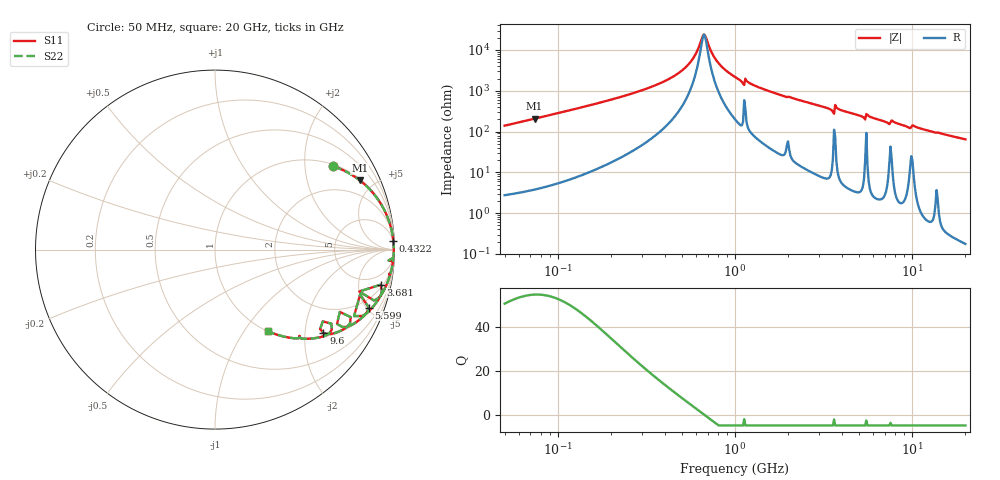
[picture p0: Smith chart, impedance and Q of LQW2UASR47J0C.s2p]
!Murata Part Number: LQW2UASR47J0C
!These Parameters are Measured in Series Mode Connection
!  o--[Z]--o
!Port1  Port2
!  o-------o
!Freq. Start=50[MHz] Stop=20[GHz], 401[Steps]
# Hz S RI R 50
!Freq.(Hz) S11(Real) S11(Imag) S21(Real) S21(Imag) S12(Real) S12(Imag) S22(Real) S22(Imag)
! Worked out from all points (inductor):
!   401 points, 50 MHz to 20 GHz, reference 50 ohm
!   read as one part in series: L = 442 nH near 51.52 MHz
!   highest Q = 54.7 at 73.81 MHz (marker M1), where L = 447 nH
!   self-resonance near 667.4 MHz
!   S11 on the Smith chart (normalised r, x): 50 MHz: 1.06, +2.79; 432.2 MHz: 5, +41; 3.681 GHz: 2.47, -8.87; 5.599 GHz: 1.30, -5.18; 9.6 GHz: 1.13, -2.49; 20 GHz: 1.00, -1.29
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5e7  0.6582 0.4646  0.3418 -0.4646  0.3418 -0.4646  0.6582 0.4646
7.380808e7  0.8069 0.3857  0.1931 -0.3857  0.1931 -0.3857  0.8069 0.3857
1.364002e8  0.9352 0.2357  0.0648 -0.2357  0.0648 -0.2357  0.9352 0.2357
3.721004e8  0.9913 0.0661  0.00867 -0.0661  0.00867 -0.0661  0.9913 0.0661
4.322267e8  0.9935 0.0481  0.00654 -0.0481  0.00654 -0.0481  0.9935 0.0481
5.575697e8  0.9955 0.0196  0.00454 -0.0196  0.00454 -0.0196  0.9955 0.0196
6.673612e8  0.9959 0.000224  0.00413 -0.000224  0.00413 -0.000224  0.9959 0.000224
7.987718e8  0.9955 -0.0192  0.00449 0.0192  0.00449 0.0192  0.9955 -0.0192
1e9  0.9938 -0.0452  0.00623 0.0452  0.00623 0.0452  0.9938 -0.0452
1.094034e9  0.9912 -0.0594  0.00875 0.0594  0.00875 0.0594  0.9912 -0.0594
1.179116e9  0.9918 -0.0593  0.00823 0.0593  0.00823 0.0593  0.9918 -0.0593
1.567309e9  0.9856 -0.1007  0.0144 0.1007  0.0144 0.1007  0.9856 -0.1007
2.728004e9  0.9552 -0.197  0.0448 0.197  0.0448 0.197  0.9552 -0.197
3.519108e9  0.9091 -0.2711  0.0909 0.2711  0.0909 0.2711  0.9091 -0.2711
3.680849e9  0.9235 -0.1955  0.0765 0.1955  0.0765 0.1955  0.9235 -0.1955
5.273168e9  0.8343 -0.3621  0.1657 0.3621  0.1657 0.3621  0.8343 -0.3621
5.598765e9  0.8567 -0.3228  0.1433 0.3228  0.1433 0.3228  0.8567 -0.3228
7.442007e9  0.6799 -0.4141  0.3201 0.4141  0.3201 0.4141  0.6799 -0.4141
7.901521e9  0.7416 -0.4247  0.2584 0.4247  0.2584 0.4247  0.7416 -0.4247
9.600142e9  0.6041 -0.4637  0.3959 0.4637  0.3959 0.4637  0.6041 -0.4637
1.034674e10  0.6391 -0.4633  0.3609 0.4633  0.3609 0.4633  0.6391 -0.4633
2e10  0.2947 -0.4545  0.7053 0.4545  0.7053 0.4545  0.2947 -0.4545
